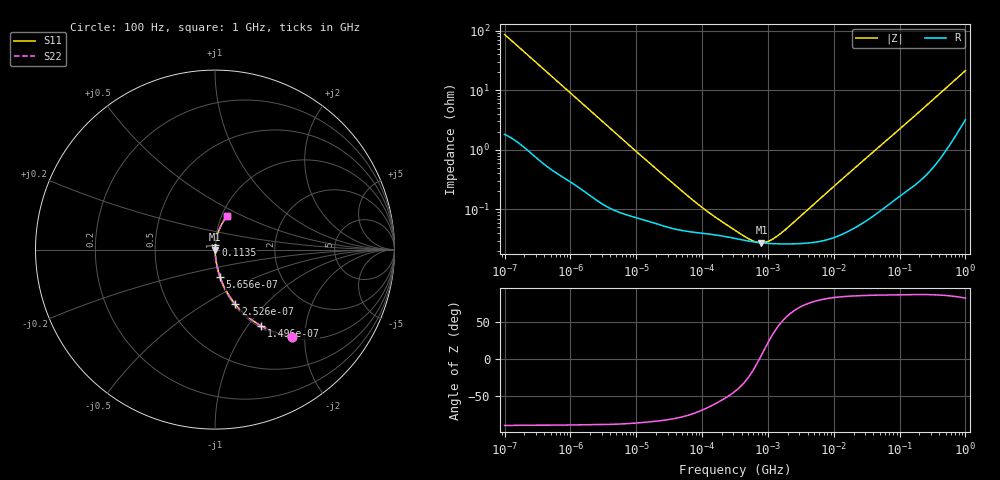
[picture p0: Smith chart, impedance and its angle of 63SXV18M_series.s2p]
!  *** S-Parameter ***
!  Copyright (C) Panasonic Industry
!  Conductive Polymer Aluminum Soild Capacitor (OS-CON)
!  Parts No. 63SXV18M
!  Connection Mode : Series
!  1  o---||---o  2
!  GND o--------o GND
!  Conditions : Temperature = 20 degC  DC Bias = 0 V
! Frequency Range : 100Hz  -  1GHz  [ 401 Steps ]
# Hz S RI R 50
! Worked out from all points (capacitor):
!   401 points, 100 Hz to 1 GHz, reference 50 ohm
!   read as one part in series: C = 18.4 uF near 108.4 Hz
!   lowest |Z| = 27.6 mohm at 798.9 kHz (marker M1)
!   series resonance near 743.1 kHz, so ESL is about 2.5 nH
!   S11 on the Smith chart (normalised r, x): 100 Hz: 1.04, -1.72; 149.6 Hz: 1.03, -1.16; 252.6 Hz: 1.02, -0.69; 565.6 Hz: 1.01, -0.31; 113.5 MHz: 1.00, +0.05; 1 GHz: 1.06, +0.42
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100  0.4275 -0.4843  0.5725 0.4843  0.5725 0.4843  0.4275 -0.4843
149.6236  0.2568 -0.425  0.7432 0.425  0.7432 0.425  0.2568 -0.425
190.5461  0.1792 -0.3713  0.8208 0.3713  0.8208 0.3713  0.1792 -0.3713
252.6388  0.1134 -0.3048  0.8866 0.3048  0.8866 0.3048  0.1134 -0.3048
363.0781  0.0608 -0.2264  0.9392 0.2264  0.9392 0.2264  0.0608 -0.2264
565.5878  0.0279 -0.1516  0.9721 0.1516  0.9721 0.1516  0.0279 -0.1516
1487.647  0.00578 -0.0601  0.9942 0.0601  0.9942 0.0601  0.00578 -0.0601
4415.704  0.00142 -0.0208  0.9986 0.0208  0.9986 0.0208  0.00142 -0.0208
22130.95  0.000574 -0.00432  0.9994 0.00432  0.9994 0.00432  0.000574 -0.00432
98287.89  0.000399 -0.00102  0.9996 0.00102  0.9996 0.00102  0.000399 -0.00102
316227.8  0.000325 -0.000305  0.9997 0.000305  0.9997 0.000305  0.000325 -0.000305
555904.3  0.000289 -0.0001  0.9997 0.0001  0.9997 0.0001  0.000289 -0.0001
679986  0.00028 -3.09e-05  0.9997 3.09e-05  0.9997 3.09e-05  0.00028 -3.09e-05
798913.9  0.000274 2.55e-05  0.9997 -2.55e-05  0.9997 -2.55e-05  0.000274 2.55e-05
1017419  0.000268 0.000114  0.9997 -0.000114  0.9997 -0.000114  0.000268 0.000114
1404430  0.000264 0.000244  0.9997 -0.000244  0.9997 -0.000244  0.000264 0.000244
4704354  0.000278 0.00112  0.9997 -0.00112  0.9997 -0.00112  0.000278 0.00112
6.99842e7  0.00147 0.0157  0.9985 -0.0157  0.9985 -0.0157  0.00147 0.0157
1.135011e8  0.00244 0.0249  0.9976 -0.0249  0.9976 -0.0249  0.00244 0.0249
3.651741e8  0.0119 0.077  0.9881 -0.077  0.9881 -0.077  0.0119 0.077
7.852356e8  0.0455 0.1556  0.9545 -0.1556  0.9545 -0.1556  0.0455 0.1556
1e9  0.0695 0.1895  0.9305 -0.1895  0.9305 -0.1895  0.0695 0.1895
